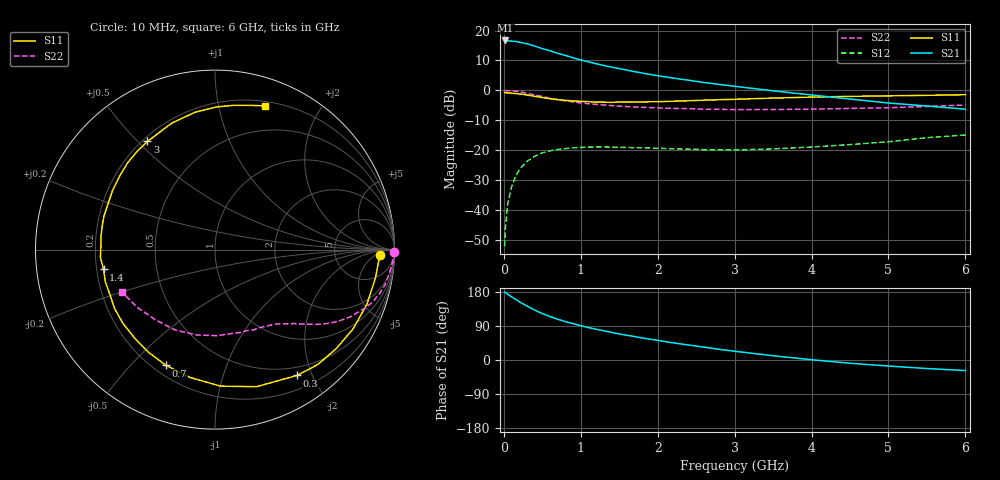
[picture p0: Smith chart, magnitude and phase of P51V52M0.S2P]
! SIEMENS Small Signal Semiconductors
! BFP183
! Si NPN RF Bipolar Junction Transistor in SOT143
! VCE = 1.5 V  IC = 2 mA
! Common Emitter S-Parameters:  March  1996
# GHz  S  MA  R  50
!  f  S11  S21  S12  S22
! GHz  MAG  ANG  MAG  ANG  MAG  ANG  MAG  ANG
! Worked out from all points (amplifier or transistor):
!   36 points, 10 MHz to 6 GHz, reference 50 ohm
!   highest |S21| = 16.7 dB at 20 MHz (marker M1)
!   |S21| within 3 dB of that: start of sweep to 537.1 MHz
!   unconditionally stable (mu >= 1): 2.058 GHz to end of sweep
!   at 250 MHz: K = 0.13, MSG = 20.4 dB, |S12| = -25.0 dB
!   at 1.4 GHz: K = 0.69, MSG = 13.4 dB, |S12| = -18.9 dB
!   at 6 GHz: K = 1.01, MAG = 3.8 dB, |S12| = -14.9 dB
!   S11 on the Smith chart (normalised r, x): 10 MHz: 20, -8; 300 MHz: 0.38, -1.78; 700 MHz: 0.25, -0.63; 1.4 GHz: 0.23, -0.08; 3 GHz: 0.22, +0.53; 6 GHz: 0.24, +1.37
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0.01  0.918 -2.0  6.768 179.0  0.0025 82.3  0.9979 -0.7
0.02  0.9138 -4.2  6.831 178.0  0.005 91.3  0.9891 -1.6
0.05  0.9078 -10.0  6.785 173.4  0.0128 86.2  0.9918 -4.0
0.1  0.8995 -19.8  6.633 166.8  0.0243 78.8  0.9803 -7.7
0.15  0.8871 -29.8  6.599 160.2  0.0361 73.2  0.9676 -11.7
0.2  0.8722 -39.2  6.411 153.9  0.0468 67.5  0.9482 -15.1
0.3  0.837 -56.9  6.028 142.5  0.0653 58.4  0.895 -21.4
0.4  0.7979 -73.2  5.501 131.7  0.0793 50.2  0.8409 -26.5
0.5  0.7613 -87.7  4.981 122.5  0.0906 43.1  0.7906 -30.5
0.6  0.7261 -101.0  4.6 114.6  0.0981 37.5  0.7437 -33.7
0.7  0.7005 -112.9  4.162 107.6  0.1033 32.4  0.7027 -36.4
0.8  0.6817 -123.1  3.838 101.3  0.1067 28.2  0.6689 -38.5
0.9  0.6668 -131.7  3.504 95.9  0.11 24.8  0.6414 -40.3
1.1  0.6487 -149.6  3.003 85.5  0.1129 19.3  0.5996 -43.4
1.4  0.6306 -169.9  2.451 72.9  0.1132 13.2  0.5582 -48.0
1.8  0.6423 167.7  1.95 58.2  0.1101 9.4  0.5223 -53.6
2.2  0.6591 150.0  1.607 45.3  0.1059 8.1  0.5001 -60.5
3  0.7105 122.0  1.173 23.1  0.1015 11.5  0.4776 -76.8
3.5  0.745 108.8  0.983 11.2  0.1053 15.5  0.4798 -88.4
4.5  0.7954 89.2  0.718 -8.6  0.1245 21.1  0.5001 -116.5
5.5  0.8274 76.2  0.549 -22.5  0.162 21.3  0.5397 -143.3
6  0.8472 71.0  0.485 -27.9  0.1803 18.1  0.5702 -155.7
